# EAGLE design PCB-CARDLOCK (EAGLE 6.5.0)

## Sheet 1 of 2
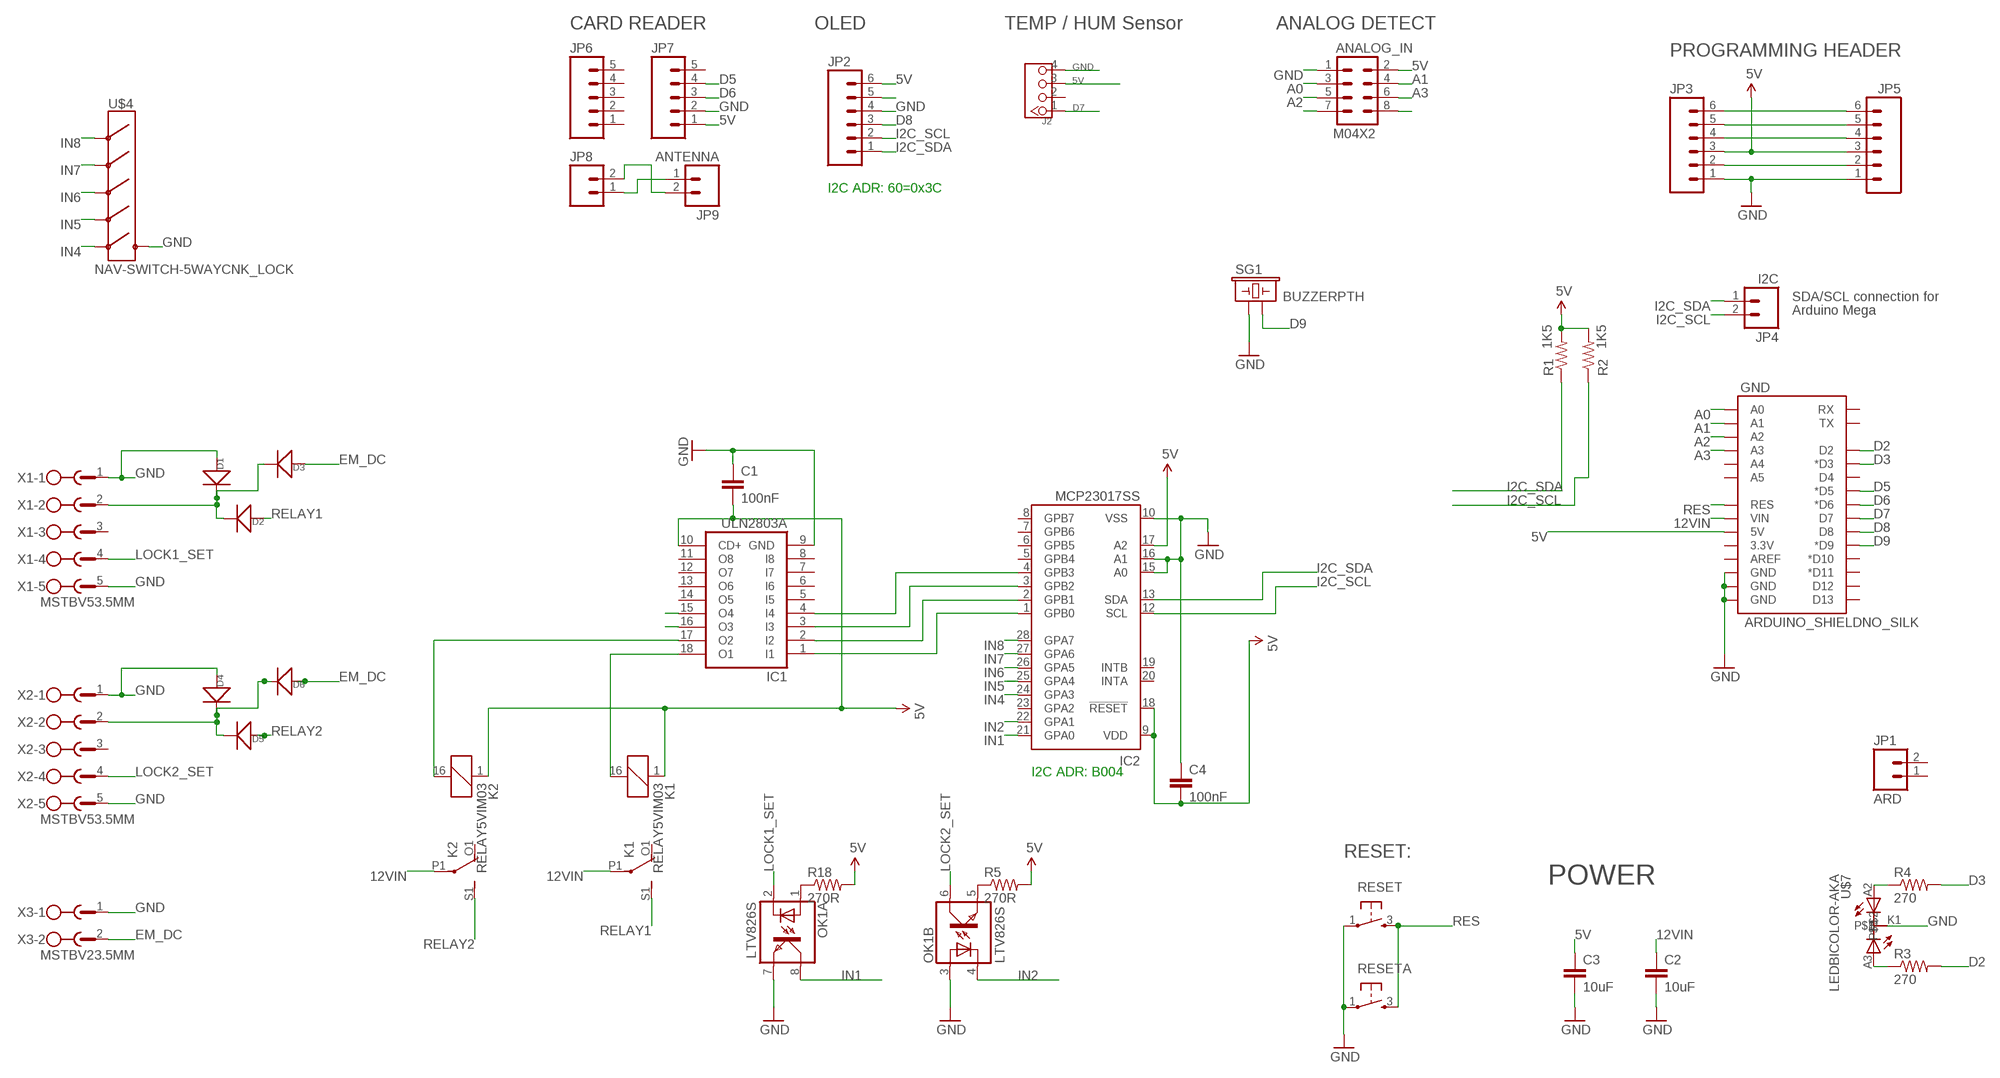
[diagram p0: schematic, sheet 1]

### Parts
ANALOG_IN  M04X2  [2X4]
C1  100nF  CAP0805  [0805]
C2  10uF  CAP0805  [0805]
C3  10uF  CAP0805  [0805]
C4  100nF  CAP0603-CAP  [0603-CAP]
D1  D-SMA  [DO-214AC]
D2  D-SMA  [DO-214AC]
D3  D-SMA  [DO-214AC]
D4  D-SMA  [DO-214AC]
D5  D-SMA  [DO-214AC]
D6  D-SMA  [DO-214AC]
GND  ARDUINO_SHIELDNO_SILK  [DUEMILANOVE_VIAS]
IC1  ULN2803A  ULN2803ASO18W  [SO18W]
IC2  MCP23017SS  [SSOP28]
J2  TWIG-4P-2.0-2.0  [4P-2.0]
JP1  ARD  M02PTH  [1X02]
JP2  M06POLAR  [MOLEX-1X6]
JP3  M06POLAR  [MOLEX-1X6]
JP4  I2C  M02PTH  [1X02]
JP5  M06POLAR  [MOLEX-1X6]
JP6  M05PTH  [1X05]
JP7  M05PTH  [1X05]
JP8  M02PTH  [1X02]
JP9  ANTENNA  M02PTH  [1X02]
K1  RELAY5VIM03  [DS2Y]
K2  RELAY5VIM03  [DS2Y]
OK1  LTV826S  [DIL8-SMD]
R1  1K5  RESISTOR0603-RES  [0603-RES]
R2  1K5  RESISTOR0603-RES  [0603-RES]
R3  270  RESISTOR0603-RES  [0603-RES]
R4  270  RESISTOR0603-RES  [0603-RES]
R5  270R  RESISTOR0603-RES  [0603-RES]
R18  270R  RESISTOR0603-RES  [0603-RES]
RESET  TAC_SWITCH  [PUSHBUTTON]
RESETA  TAC_SWITCH  [PUSHBUTTON]
SG1  BUZZERPTH  [BUZZER-12MM]
U$4  NAV-SWITCH-5WAYCNK_LOCK  [NAV-SWITCH-5WAY]
U$7  LEDBICOLOR-AKA  [LED5MM-BICOLOR]
X1  MSTBV53.5MM  [MSTBV5-3.5]
X2  MSTBV53.5MM  [MSTBV5-3.5]
X3  MSTBV23.5MM  [MSTBV2-3.5]

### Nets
5V [PWR]: ANALOG_IN.2 C1.2 C3.1 C4.2 GND.5V IC1.10(CD+) IC2.9(VDD) IC2.17(A2) IC2.18(!RESET) J2.3 JP2.6 JP3.3 JP5.3 JP7.1 K1.1 K2.1 R1.2 R2.2 R5.2 R18.2
12VIN [PWR]: C2.1 GND.VIN K1.P1(2:P) K2.P1(2:P)
A0: ANALOG_IN.3 GND.A0
A1: ANALOG_IN.4 GND.A1
A2: ANALOG_IN.5 GND.A2
A3: ANALOG_IN.6 GND.A3
D2: GND.D2 R3.2
D3: GND.D3(*D3) R4.2
D5: GND.D5(*D5) JP7.4
D6: GND.D6(*D6) JP7.3
D7: GND.D7 J2.1
D8: GND.D8 JP2.3
D9: GND.D9(*D9) SG1.-
EM_DC [RELAY LINES]: D3.1(+) D6.1(+) X3.2
GND [PWR]: ANALOG_IN.1 C1.1 C2.2 C3.2 C4.1 D1.1(+) D4.1(+) GND.GND@0(GND) GND.GND@1(GND) GND.GND@2(GND) IC1.9(GND) IC2.10(VSS) IC2.15(A0) IC2.16(A1) J2.4 JP2.4 JP3.1 JP5.1 JP7.2 OK1.3(B:A) OK1.7(A:EMIT) RESET.1 RESETA.1 SG1.+ U$4.PIN4(COMMON) U$7.K1 X1.1 X1.5 X2.1 X2.5 X3.1
I2C_SCL: IC2.12(SCL) JP2.2 JP4.2 R2.1
I2C_SDA: IC2.13(SDA) JP2.1 JP4.1 R1.1
IN1: IC2.21(GPA0) OK1.8(A:COL)
IN2: IC2.22(GPA1) OK1.4(B:C)
IN4: IC2.24(GPA3) U$4.PIN6(PUSH)
IN5: IC2.25(GPA4) U$4.PIN5(RIGHT)
IN6: IC2.26(GPA5) U$4.PIN2(LEFT)
IN7: IC2.27(GPA6) U$4.PIN3(DWN)
IN8: IC2.28(GPA7) U$4.PIN1(UP)
LOCK1_SET [PWR]: OK1.2(A:C) X1.4
LOCK2_SET [PWR]: OK1.6(B:COL) X2.4
N$1 [RELAY LINES]: D1.2(-) D2.2(-) D3.2(-) X1.2
N$2: JP8.1 JP9.1
N$3: JP3.4 JP5.4
N$4: IC1.18(O1) K1.16
N$5 [RELAY LINES]: D4.2(-) D5.2(-) D6.2(-) X2.2
N$6: IC1.1(I1) IC2.1(GPB0)
N$7: R4.1 U$7.A2
N$8: JP3.5 JP5.5
N$9: IC1.17(O2) K2.16
N$10: JP8.2 JP9.2
N$11: R3.1 U$7.A3
N$12: JP3.2 JP5.2
N$13: IC1.2(I2) IC2.2(GPB1)
N$14: IC1.3(I3) IC2.3(GPB2)
N$15: JP2.5
N$16: IC1.4(I4) IC2.4(GPB3)
N$17: ANALOG_IN.8
N$18: OK1.5(B:EMIT) R5.1
N$21: ANALOG_IN.7
N$23: OK1.1(A:A) R18.1
N$25: IC1.16(O3)
N$26: IC1.15(O4)
N$45: JP3.6 JP5.6
RELAY1 [RELAY LINES]: D2.1(+) K1.S1(2:S)
RELAY2 [RELAY LINES]: D5.1(+) K2.S1(2:S)
RES: GND.RES RESET.3 RESETA.3
Unconnected: GND.3.3V GND.A4 GND.A5 GND.AREF GND.D4 GND.D10(*D10) GND.D11(*D11) GND.D12 GND.D13 GND.RX GND.TX IC1.5(I5) IC1.6(I6) IC1.7(I7) IC1.8(I8) IC1.11(O8) IC1.12(O7) IC1.13(O6) IC1.14(O5) IC2.5(GPB4) IC2.6(GPB5) IC2.7(GPB6) IC2.8(GPB7) IC2.19(INTB) IC2.20(INTA) IC2.23(GPA2) J2.2 JP1.1 JP1.2 JP6.1 JP6.2 JP6.3 JP6.4 JP6.5 JP7.5 K1.O1(2:O) K1.O2(3:O) K1.P2(3:P) K1.S2(3:S) K2.O1(2:O) K2.O2(3:O) K2.P2(3:P) K2.S2(3:S) X1.3 X2.3

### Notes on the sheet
- CARD READER | OLED | TEMP / HUM Sensor | ANALOG DETECT
- PROGRAMMING HEADER
- I2C ADR: 60=0x3C
- SDA/SCL connection for
- Arduino Mega
- I2C ADR: B004
- RESET:
- POWER

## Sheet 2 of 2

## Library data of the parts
ANALOG_IN = SparkFun:M04X2
C1-C4 = SparkFun:CAP: Capacitor
D1-D6 = OPL:D*: DIODE
GND = SparkFun:ARDUINO_SHIELD
IC1 = uln-udn:ULN2803A: DRIVER ARRAY
IC2 = microchip:MCP23017: http://ww1.microchip.com/downloads/en/DeviceDoc/21952a.pdf Source: http://ww1.microchip.com/downloads/en/DeviceDoc/21952a.pdf; MF: MICROCHIP; MPN: MCP23017-E/SS; OC_FARNELL: 1467674; OC_NEWARK: 31K2960
J2 = Connector :TWIG-4P-2.0
JP1 JP4 JP8 JP9 = SparkFun:M02: Header 2
JP2 JP3 JP5 = SparkFun:M06: Header 6 Standard 6-pin 0.1" header. Use with straight break away headers (SKU : PRT-00116), right angle break away headers (PRT-00553), swiss pins (PRT-00743), machine pins (PRT-00117), and female headers (PRT-00115). Molex polarized connector foot print use with SKU : PRT-08094 with associated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
JP6 JP7 = SparkFun:M05: Header 5 Standard 5-pin 0.1" header. Use with straight break away headers (SKU : PRT-00116), right angle break away headers (PRT-00553), swiss pins (PRT-00743), machine pins (PRT-00117), and female headers (PRT-00115). Molex polarized connector foot print use with SKU : PRT-08230 with associated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
K1 K2 = SKAARHOJ:RELAY5V: RELAY 2 x switch, AxiCom 150 mW 5V
OK1 = optocoupler:LTV826: OPTO COUPLER Source: LITEON, LTV816.pdf; OC_FARNELL: unknown; OC_NEWARK: unknown
R1-R5 R18 = SparkFun:RESISTOR: Resistor
RESET RESETA = SKAARHOJ:TAC_SWITCH: Momentary Switch
SG1 = SparkFun:BUZZER: Buzzer 12mm
U$4 = SKAARHOJ:NAV-SWITCH-5WAY: For use with a push-button switch made by CnK components. The Part # is
U$7 = SKAARHOJ:LEDBICOLOR-AKA
X1 X2 = SKAARHOJ:MSTBV5: PHOENIX
X3 = SKAARHOJ:MSTBV2: PHOENIX

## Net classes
0 default: width 0.203 mm, drill 0.406 mm, clearance 0.203 mm
1 PWR: width 0.406 mm, drill 0.61 mm, clearance 0.203 mm
2 RELAY LINES: width 0.305 mm, clearance 0.203 mm
3 INput lines: clearance 0.203 mm

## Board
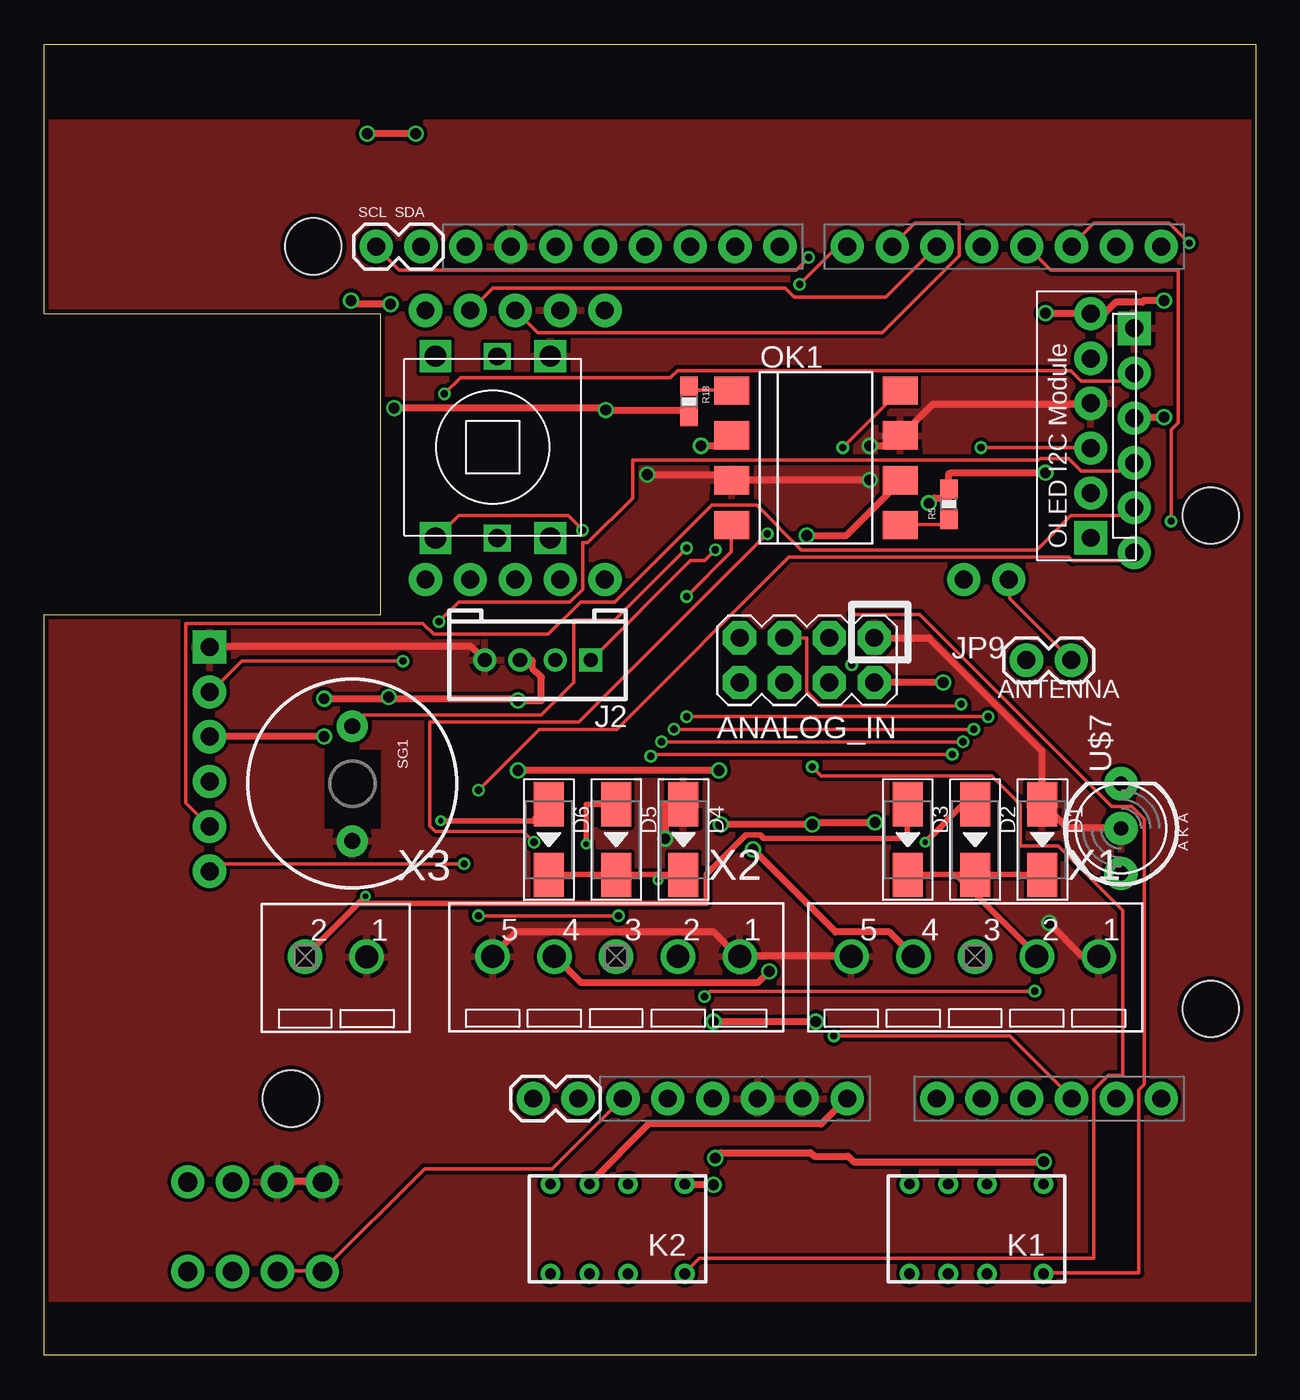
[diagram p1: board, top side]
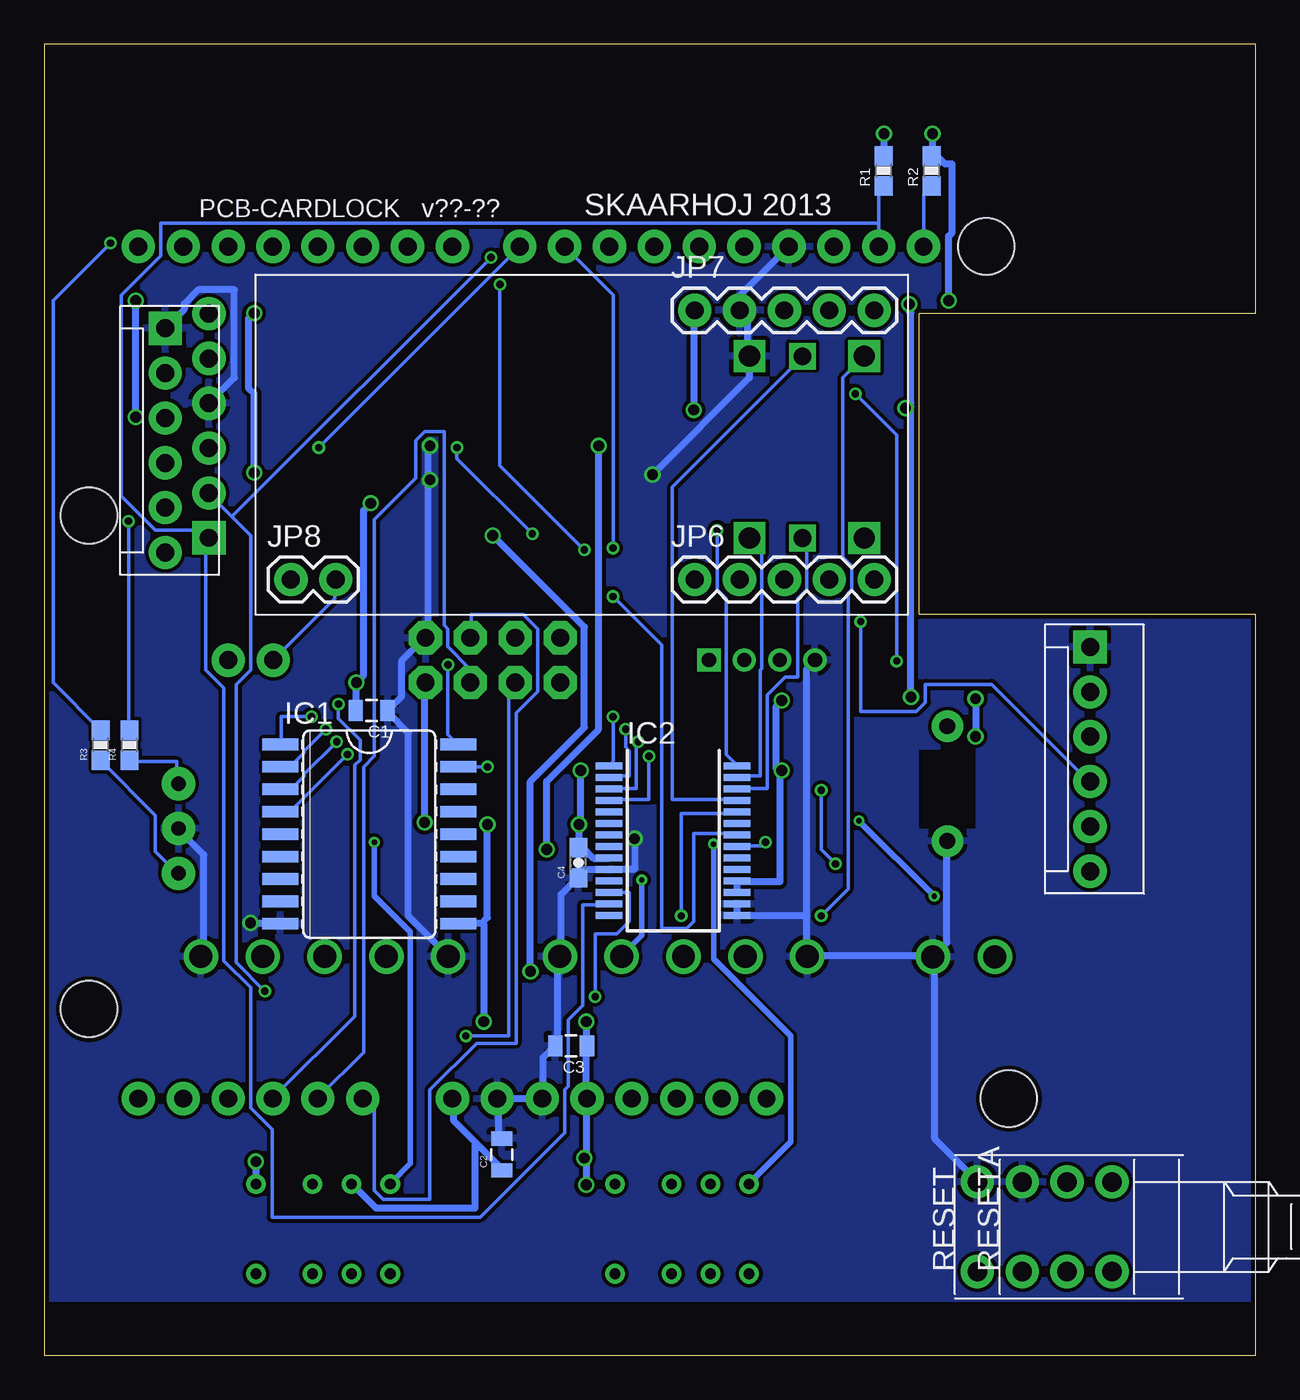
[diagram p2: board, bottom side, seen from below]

Size 68.58 x 74.26 mm. Coordinates in mm from the lower left corner, seen from the top.
Outline: 0,0 0,41.96 19.05,41.96 19.05,58.99 0,58.99 0,74.26 68.58,74.26 68.58,0 0,0
Copper layers (1*16): Top 0.035mm / dielectric 1.5mm / Bottom 0.035mm
Design rules "Fusion_eagle_rule_v1.1": minimum track width 6mil, minimum drill 12mil, track to track 6mil, track to pad 6mil, pad to pad 6mil, via to via 6mil, smd to smd 0mil, copper to edge 10mil, drill to drill 10mil, minimum pad ring 10mil, minimum via ring 6mil, stop-mask expansion 2mil, vias tented up to drill 100mil, thermal gap 10mil
Holes 3.2 mm at 66.04,47.56 15.24,62.8 13.97,14.54 66.04,19.62
tRestrict: area 0,0 to 68.6,3; area 0,70 to 68.6,74; area 15.9,29.8 to 19,34.3
bRestrict: area 0,70 to 68.6,74; area 0,0 to 68.6,3; area 15.9,29.8 to 19,34.3

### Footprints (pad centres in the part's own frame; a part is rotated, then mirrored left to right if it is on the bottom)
2X4 = drill 1.016 pad 1.88 octagon: 1 -3.81,-1.27; 2 -3.81,1.27; 3 -1.27,-1.27; 4 -1.27,1.27; 5 1.27,-1.27; 6 1.27,1.27; 7 3.81,-1.27; 8 3.81,1.27
0805 = smd 0.8 x 1.2: 1 -0.9,0; 2 0.9,0
0603-CAP = smd 1.1 x 1: 1 -0.85,0; 2 0.85,0
DO-214AC = smd 2.5 x 1.7: 1 -2,0; 2 2,0
DUEMILANOVE_VIAS = drill 1.016 pad 1.88: 3.3V 50.8,13.97; 5V 50.8,16.51; A0 50.8,29.21; A1 50.8,31.75; A2 50.8,34.29; A3 50.8,36.83; A4 50.8,39.37; A5 50.8,41.91; AREF 2.54,2.54; D2 2.54,36.83; D3 2.54,34.29; D4 2.54,31.75; D5 2.54,29.21; D6 2.54,26.67; D7 2.54,24.13; D8 2.54,20.32; D9 2.54,17.78; D10 2.54,15.24; D11 2.54,12.7; D12 2.54,10.16; D13 2.54,7.62; GND@0 50.8,19.05; GND@1 50.8,21.59; GND@2 2.54,5.08; RES 50.8,11.43; RX 2.54,41.91; TX 2.54,39.37; VIN 50.8,24.13
SO18W = smd 0.66 x 2.032: 1 -5.08,-5.029; 2 -3.81,-5.029; 3 -2.54,-5.029; 4 -1.27,-5.029; 5 0,-5.029; 6 1.27,-5.029; 7 2.54,-5.029; 8 3.81,-5.029; 9 5.08,-5.029; 10 5.08,5.029; 11 3.81,5.029; 12 2.54,5.029; 13 1.27,5.029; 14 0,5.029; 15 -1.27,5.029; 16 -2.54,5.029; 17 -3.81,5.029; 18 -5.08,5.029
SSOP28 = smd 0.4 x 1.5: 1 -4.225,-3.625; 2 -3.575,-3.625; 3 -2.925,-3.625; 4 -2.275,-3.625; 5 -1.625,-3.625; 6 -0.975,-3.625; 7 -0.325,-3.625; 8 0.325,-3.625; 9 0.975,-3.625; 10 1.625,-3.625; 11 2.275,-3.625; 12 2.925,-3.625; 13 3.575,-3.625; 14 4.225,-3.625; 15 4.225,3.625; 16 3.575,3.625; 17 2.925,3.625; 18 2.275,3.625; 19 1.625,3.625; 20 0.975,3.625; 21 0.325,3.625; 22 -0.325,3.625; 23 -0.975,3.625; 24 -1.625,3.625; 25 -2.275,3.625; 26 -2.925,3.625; 27 -3.575,3.625; 28 -4.225,3.625
4P-2.0 = drill 0.8 pad 1.27 square: 1 -3,0 | drill 0.8 pad 1.27: 2 -1,0; 3 1,0; 4 3,0
1X02 = drill 1.016 pad 1.88: 1 0,0; 2 2.54,0
MOLEX-1X6 = drill 1.016 pad 1.88 square: 1 0,0 | drill 1.016 pad 1.88: 2 2.54,0; 3 5.08,0; 4 7.62,0; 5 10.16,0; 6 12.7,0
1X05 = drill 1.016 pad 1.88: 1 0,0; 2 2.54,0; 3 5.08,0; 4 7.62,0; 5 10.16,0
DS2Y = drill 0.6: 1 1.2,0.46; 16 1.2,5.54; O1 4.4,0.46; O2 4.4,5.54; P1 6.6,0.46; P2 6.6,5.54; S1 8.8,0.46; S2 8.8,5.54
DIL8-SMD = smd 1.6 x 2: 1 -3.81,-4.77; 2 -1.27,-4.77; 3 1.27,-4.77; 4 3.81,-4.77; 5 3.81,4.77; 6 1.27,4.77; 7 -1.27,4.77; 8 -3.81,4.77
0603-RES = smd 1.1 x 1: 1 -0.85,0; 2 0.85,0
PUSHBUTTON = drill 1.1 pad 1.88: 1 2.54,2.54; 2 2.54,-2.54; 3 -2.54,2.54; 4 -2.54,-2.54
BUZZER-12MM = drill 0.9 pad 1.778: + 3.25,0; - -3.25,0
NAV-SWITCH-5WAY = drill 1.2 square: PIN1 -5.15,3.25; PIN3 -5.15,-3.25; PIN4 5.15,-3.25; PIN6 5.15,3.25 | drill 1 square: PIN2 -5.15,-0.25; PIN5 5.15,-0.25
LED5MM-BICOLOR = drill 0.813 pad 1.88: A2 2.54,0; A3 -2.54,0; K1 0,0
MSTBV5-3.5 = drill 1.3: 1 -7,0; 2 -3.5,0; 3 0,0; 4 3.5,0; 5 7,0
MSTBV2-3.5 = drill 1.3: 1 -1.75,0.02; 2 1.75,0.02

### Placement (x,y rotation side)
ANALOG_IN  43.18,39.37 180 top
C1  50.04,36.52 180 bottom
C2  42.67,11.38 90 bottom
C3  38.75,17.53 180 bottom
C4  38.34,27.89 90 bottom
D1  56.52,29.21 270 top
D2  52.7,29.21 270 top
D3  48.9,29.21 270 top
D4  36.2,29.21 270 top
D5  32.38,29.21 270 top
D6  28.57,29.21 270 top
GND  21.34,65.34 270 top
IC1  50.17,29.52 270 bottom
IC2  32.97,29.14 270 bottom
J2  27.94,39.37 180 top
JP1  27.69,14.54 0 top
JP2  59.25,46.3 90 top
JP3  61.72,58.17 270 bottom
JP4  21.34,62.8 180 top
JP5  9.36,40.12 270 bottom
JP6  31.75,43.94 0 bottom
JP7  31.75,59.18 0 bottom
JP8  54.61,43.94 0 bottom
JP9  58.15,39.37 180 top
K1  57.78,10.16 180 top
K2  37.47,10.16 180 top
OK1  43.7,50.83 270 top
R1  21.05,67.09 90 bottom
R2  18.33,67.09 90 bottom
R3  65.38,34.56 90 bottom
R4  63.74,34.56 90 bottom
R5  51.23,48.21 90 top
R18  36.5,54.02 270 top
RESET  13.21,7.29 90 bottom
RESETA  10.67,7.29 90 bottom
SG1  17.45,32.38 270 top
U$4  25.4,51.44 90 top
U$7  60.97,29.84 90 top
X1  52.7,22.59 180 top
X2  32.38,22.59 180 top
X3  16.51,22.59 180 top

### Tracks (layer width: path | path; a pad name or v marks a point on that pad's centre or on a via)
5V  (via drill 0.61)
  Top 0.406: v63.4,59.74 62.28,59.74 62.18,59.64 60.66,59.64 60.05,59.03 59.33,59.03 JP2.6 59.13,59.03 v56.69,59.03 | v63.4,53.14 61.77,53.14 JP3.3 | v50.9,38.1 ANALOG_IN.2 | v50.09,48.26 50.39,48.56 51.21,48.56 51.21,48.97 R5.2 51.21,49.17 51.21,49.89 51.31,49.99 v56.69,49.99 | v21.03,69.19 v18.29,69.19 | R18.2 36.47,53.24 36.47,53.54 v31.8,53.54 31.7,53.65 v19.81,53.65 | v17.37,59.74 17.58,59.54 v19.61,59.54 | v37.9,9.65 36.27,9.65 K2.1 | v56.59,10.97 45.82,10.97 45.52,11.28 43.59,11.28 43.38,11.48 38.3,11.48 v38,11.18 | v38.3,30.07 v43.48,30.07 43.59,30.18 v47.04,30.18 | v38.2,33.12 v26.82,33.12 | J2.3 27.03,39.42 27.53,39.42 27.64,39.32 27.64,38.91 28.14,38.41 28.14,37.08 v26.82,37.08 26.72,37.19 19.51,37.19 | v15.85,35.05 9.45,35.05 JP5.3 | 19.51,37.19 v15.85,37.19 | v43.69,18.9 v37.9,18.9 | v19.51,37.29 19.51,37.19
  Bottom 0.406: v63.4,53.14 v63.4,59.74 | C1.2 50.9,36.58 v50.9,38.1 50.49,38.51 50.49,47.85 v50.09,48.26 | v56.69,59.03 57,58.73 57,54.76 56.69,54.46 v56.69,49.99 | v18.29,69.19 18.29,67.97 R2.2 18.09,67.97 17.58,67.46 17.17,67.46 17.17,63.6 17.37,63.4 v17.37,59.74 | v21.03,69.19 21.03,67.97 R1.2 | v31.8,53.54 31.8,59.13 JP7.1 | v19.61,59.54 19.61,59.13 19.51,59.03 19.51,53.95 v19.81,53.65 19.51,53.75 v19.51,37.29 | 37.9,11.18 37.9,14.43 GND.5V 37.9,14.63 37.9,17.48 C3.1 37.9,17.68 v37.9,18.9 | 37.9,11.18 v37.9,9.65 | v56.59,10.97 56.59,9.75 K1.1 | v38,11.18 37.9,11.18 | IC2.17 29.36,26.31 29.36,26.82 IC2.18 29.16,26.82 26.92,26.82 26.92,33.02 v26.82,33.12 27.03,33.12 27.13,33.22 27.13,36.78 v26.82,37.08 | v43.48,30.07 43.48,24.79 43.79,24.49 | 43.79,24.49 45.11,24.49 IC1.10 | IC2.9 36.68,28.14 37.49,28.14 38.1,28.75 C4.2 38.3,28.75 v38.3,30.07 38.2,30.18 v38.2,33.12 | v15.85,37.19 v15.85,35.05 | v43.69,18.9 43.69,24.38 43.79,24.49 | v47.04,30.18 47.04,38.1 ANALOG_IN.2
12VIN
  Top 0.406: K2.P1 30.89,9.75 34.24,13.11 43.99,13.11 45.41,14.53 GND.VIN
  Bottom 0.406: 44.09,11.99 45.41,13.31 45.41,14.53 GND.VIN | 44.09,11.99 42.67,10.57 C2.1 | K1.P1 51.1,9.65 49.78,8.33 44.2,8.33 44.2,11.89 44.09,11.99
A0
  Bottom 0.203: GND.A0 50.49,14.53 49.89,13.92 49.89,9.35 49.38,8.84 46.74,8.84 46.74,15.04 44.09,17.68 41.86,17.68 41.86,36.37 40.64,37.59 40.64,41.15 41.45,41.96 44.4,41.96 44.4,40.64 ANALOG_IN.3
A1
  Bottom 0.203: GND.A1 53.03,14.63 50.49,17.17 50.49,33.33 49.89,33.93 49.89,47.35 47.55,49.68 47.55,51.82 47.04,52.32 45.92,52.32 45.92,41.35 45.72,41.15 45.72,40.13 44.5,38.91 44.5,38.1 ANALOG_IN.4
A2  (via drill 0.41)
  Top 0.203: v51.92,36.88 51.82,36.78 43.99,36.78 43.18,37.59 43.18,40.64 ANALOG_IN.5
  Bottom 0.203: v51.92,36.88 51.92,36.07 50.7,34.85 50.7,33.73 51,33.43 51,19.2 55.58,14.63 GND.A2
A3  (via drill 0.41)
  Top 0.203: v44.7,18.09 54.66,18.09 58.12,14.63 GND.A3
  Bottom 0.203: v44.7,18.09 42.27,18.09 42.27,37.8 41.96,38.1 ANALOG_IN.6
D2  (via drill 0.41)
  Top 0.203: v64.82,62.99 63.7,64.11 59.44,64.11 58.22,62.89 GND.D2
  Bottom 0.203: v64.82,62.99 68.07,59.74 68.07,38.1 65.43,35.46 R3.2
D3  (via drill 0.41)
  Top 0.203: v63.8,47.24 63.8,52.43 64.21,52.83 64.21,61.47 57,61.47 55.68,62.79 GND.D3
  Bottom 0.203: v63.8,47.24 63.8,35.46 R4.2
D5
  Top 0.203: JP7.4 25.4,60.45 41.96,60.45 42.47,59.94 47.65,59.94 50.49,62.79 GND.D5
D6
  Top 0.203: JP7.3 27.94,57.91 47.45,57.91 51.82,62.28 51.82,64.11 49.28,64.11 48.06,62.89 GND.D6
D7  (via drill 0.41)
  Top 0.203: v38,45.62 37.39,45.01 36.58,45.01 30.99,39.42 J2.1 | v42.77,60.66 44.91,62.79 45.41,62.79 GND.D7
  Bottom 0.203: v38,45.62 42.77,50.39 v42.77,60.66
D8  (via drill 0.41)
  Top 0.203: v53.03,51.41 59.23,51.41 JP2.3
  Bottom 0.203: v53.03,51.41 GND.D8
D9  (via drill 0.41)
  Top 0.203: v36.37,45.72 32.31,41.66 29.97,41.66 29.97,38.1 28.14,36.27 18.09,36.27 17.48,35.66 SG1.-
  Bottom 0.203: v36.37,45.72 36.37,60.05 GND.D9
EM_DC  (via drill 0.3)
  Top 0.305: v22.45,30.28 27.64,30.28 28.55,31.19 D6.1 | 17.88,25.7 14.83,22.66 X3.2 | 17.88,25.7 v18.19,26.01 | D3.1 48.87,31.19 48.87,29.26 40.74,29.26 40.54,29.46 39.73,29.46 37.49,27.23 37.49,25.6 17.98,25.6 17.88,25.7
  Bottom 0.305: v18.19,26.01 v22.45,30.28
GND  (via drill 0.61)
  Top 0.406: RESETA.1 13.21,9.86 15.75,9.86 RESET.1 | JP5.1 9.45,40.13 24.18,40.13 24.89,39.42 J2.4 | v34.14,49.89 38.61,49.89 38.91,49.58 OK1.3 39.12,49.58 v46.74,49.58 | JP2.4 59.23,53.85 50.29,53.85 48.56,52.12 OK1.7 48.26,52.12 47.65,51.51 v46.74,51.51 | U$7.K1 60.96,29.87 57.91,29.87 56.59,31.19 D1.1 56.49,31.39 56.49,34.24 50.09,40.64 ANALOG_IN.1 | v56.9,24.49 58.73,22.66 59.64,22.66 X1.1 | v35.15,29.26 35.15,31.19 36.17,31.19 D4.1 | X1.5 45.62,22.66 39.42,22.66 X2.1 39.22,22.66 37.9,23.98 26.72,23.98 25.4,22.66 X2.5
  Bottom 0.406: SG1.+ 17.48,29.06 17.48,23.37 18.19,22.66 X3.1 | RESET.1 15.75,9.86 18.19,12.29 18.19,22.45 X3.1 | IC2.16 29.36,25.5 29.36,24.99 IC2.15 29.16,24.89 25.4,24.89 | 25.4,24.89 25.4,22.66 X2.5 25.2,22.66 18.39,22.66 X3.1 | 25.4,24.89 25.4,38.91 24.99,39.32 J2.4 | v34.14,49.89 28.65,55.37 28.65,56.49 U$4.PIN4 28.75,56.69 28.75,58.73 JP7.2 29.16,59.33 29.16,60.05 GND.GND@2 | JP3.1 60.66,59.23 60.66,59.54 59.84,60.35 57.81,60.35 57.81,55.37 59.23,53.95 JP2.4 | v56.9,24.49 55.27,24.49 IC1.9 | U$7.K1 60.96,29.77 59.54,28.35 59.54,22.76 59.64,22.66 X1.1 | C2.2 42.67,12.29 42.88,12.5 42.88,14.53 GND.GND@1 42.67,14.53 40.54,14.53 GND.GND@0 40.34,14.63 40.34,16.87 39.73,17.48 C3.2 39.52,17.68 39.52,22.45 X2.1 39.32,22.66 39.32,26.11 38.41,27.03 C4.1 38.3,27.23 38.3,27.53 36.78,27.53 IC2.10 36.58,27.53 35.15,27.53 v35.15,29.26 | X1.5 45.72,22.66 47.95,24.89 47.95,35.26 49.07,36.37 C1.1 49.07,36.58 48.36,37.29 48.36,39.32 47.04,40.64 ANALOG_IN.1 46.84,40.74 46.84,49.58 | v46.74,51.51 46.84,51.41 46.84,49.58 | v46.74,49.58 46.84,49.58
  pour Top: 0,0 68.58,0 68.58,74.3 0,74.3
  pour Bottom: 0,0 68.58,0 68.58,74.3 0,74.3
I2C_SCL  (via drill 0.41)
  Top 0.203: v37.39,20.32 37.69,20.62 v56.08,20.62 | v43.28,62.18 42.57,61.47 20.12,61.47 JP4.2
  Bottom 0.203: JP4.2 18.8,65.73 18.39,66.14 R2.1 | v37.39,20.32 37.39,23.88 36.17,23.88 35.46,24.59 35.46,26.21 36.58,26.21 IC2.12 | v56.08,20.62 57.71,22.25 57.71,38 56.9,38.81 56.9,46.43 57.96,47.5 | 57.96,47.5 59.23,48.77 JP2.2 | 57.96,47.5 v43.28,62.18
I2C_SDA
  Bottom 0.203: JP4.1 21.34,64.11 | 21.34,64.11 21.34,65.94 21.13,66.14 R1.1 | IC2.13 36.68,25.5 38.1,25.5 38.1,19.81 38.91,19 38.91,15.24 39.12,15.04 39.12,12.6 43.89,7.82 55.68,7.82 55.68,12.8 56.9,14.02 56.9,20.83 58.42,22.35 58.42,37.8 59.44,38.81 59.44,46.13 59.33,46.23 JP2.1 59.33,46.33 59.33,46.74 62.28,46.74 64.21,48.67 64.21,60.05 61.98,62.28 61.98,64.11 21.34,64.11
IN1  (via drill 0.41)
  Top 0.203: v27.74,29.06 27.13,29.67 22.15,29.67 21.84,29.97 21.84,35.87 30.28,35.87 v40.95,46.53 | v45.21,51.41 48.36,54.56 48.46,54.56 OK1.8
  Bottom 0.203: v27.74,29.06 27.74,28.85 29.26,28.85 IC2.21 | v40.95,46.53 45.21,50.8 v45.21,51.41
IN2  (via drill 0.41)
  Top 0.203: v36.37,42.98 38.91,45.52 38.91,46.94 OK1.4
  Bottom 0.203: v36.37,42.98 33.63,40.23 33.63,24.18 32.21,24.18 31.8,24.59 31.8,29.57 29.36,29.57 IC2.22
IN4  (via drill 0.41)
  Top 0.203: v24.59,24.89 v32.51,24.89
  Bottom 0.203: v32.51,24.89 32.51,30.68 29.36,30.68 IC2.24 | v24.59,24.89 23.06,26.42 23.06,43.18 22.86,43.38 22.86,44.7 23.37,45.21 23.37,55.37 22.25,56.49 U$4.PIN6
IN5
  Bottom 0.203: IC2.25 29.36,31.5 33.02,31.5 33.02,49.17 25.7,56.49 U$4.PIN5
IN6
  Bottom 0.203: IC2.26 29.26,32.11 27.64,32.11 27.64,37.39 26.62,38.41 25.91,38.41 25.91,42.88 25.4,43.38 25.4,46.02 25.6,46.23 U$4.PIN2
IN7
  Bottom 0.203: IC2.27 29.26,32.82 28.04,32.82 28.04,38.81 27.94,38.91 27.94,45.62 28.55,46.23 U$4.PIN3
IN8  (via drill 0.41)
  Top 0.203: v30.48,46.74 29.67,47.55 23.47,47.55 22.25,46.33 U$4.PIN1
  Bottom 0.203: v30.48,46.74 30.48,43.38 29.97,42.88 29.97,34.04 29.36,33.43 IC2.28
LOCK1_SET  (via drill 0.61)
  Top 0.406: v37.19,51.51 38.41,51.51 38.91,52.02 OK1.2 | v40.13,28.65 44.81,23.98 47.85,23.98 49.17,22.66 X1.4
  Bottom 0.406: v37.19,51.51 37.19,35.46 40.13,32.51 v40.13,28.65
LOCK2_SET  (via drill 0.61)
  Top 0.406: v43.18,46.43 45.41,46.43 48.46,49.48 OK1.6 | v41.05,21.74 40.44,21.13 30.38,21.13 28.96,22.55 X2.4
  Bottom 0.406: v43.18,46.43 38,41.25 38,35.56 41.05,32.51 v41.05,21.74
N$1
  Top 0.305: 51.71,27.23 52.63,27.23 D2.2 52.83,27.23 56.49,27.23 D1.2 | 51.71,27.23 48.97,27.23 D3.2 | X1.2 56.19,22.66 51.71,27.13 51.71,27.23
N$2
  Top 0.203: JP9.1 58.12,39.42 54.66,42.88 54.66,43.89 JP8.1
N$3  (via drill 0.41)
  Top 0.203: v22.35,41.55 23.47,42.67 29.77,42.67 30.48,43.38 30.48,46.02 30.79,46.02 33.33,48.56 33.33,50.7 56.29,50.7 56.39,50.8 58.01,50.8 58.73,50.09 61.27,50.09 JP3.4
  Bottom 0.203: v22.35,41.55 22.35,36.47 19.2,36.47 18.69,36.98 18.69,38 14.94,38 9.45,32.51 JP5.4
N$4  (via drill 0.41)
  Top 0.203: v45.72,39.12 45.72,41.96 49.58,41.96 60.45,31.09 61.57,31.09 62.28,30.38 62.28,15.34 61.98,15.04 61.98,4.67 56.59,4.67 K1.16
  Bottom 0.203: v45.72,39.12 45.72,35.15 45.21,34.65 IC1.18
N$5  (via drill 0.3)
  Top 0.305: D6.2 28.65,27.23 32.31,27.23 D5.2 32.51,27.23 34.75,27.23 | 34.75,27.23 36.17,27.23 D4.2 | 34.75,27.23 v34.75,26.92
  Bottom 0.305: v34.75,26.92 34.75,23.77 35.87,22.66 X2.2
N$6  (via drill 0.41)
  Top 0.203: v53.44,36.17 v36.37,36.17
  Bottom 0.203: v36.37,36.17 36.37,33.63 36.58,33.43 IC2.1 | v53.44,36.17 55.17,36.17 55.17,34.65 IC1.1
N$7
  Bottom 0.203: R4.1 63.7,33.63 61.06,33.63 61.06,32.41 U$7.A2
N$8
  Top 0.203: JP3.5 61.27,47.55 58.12,47.55 56.19,45.62 42.88,45.62 40.34,48.16 37.8,48.16 32.31,42.67 30.38,42.67 28.55,40.84 22.05,40.84 21.44,41.45 8.03,41.45 8.03,31.29 9.35,29.97 JP5.5
N$9  (via drill 0.41)
  Top 0.203: v43.48,33.33 43.99,32.82 53.65,32.82 55.27,31.19 55.27,28.85 57.4,28.85 61.06,25.2 61.06,15.85 60.25,15.85 59.44,15.04 59.44,5.49 37.08,5.49 36.27,4.67 K2.16
  Bottom 0.203: v43.48,33.33 45.11,33.33 IC1.17
N$10
  Bottom 0.203: JP9.2 55.58,39.42 52.12,42.88 52.12,43.89 JP8.2
N$11
  Bottom 0.203: R3.1 65.33,33.63 62.28,30.58 62.28,28.55 61.06,27.33 U$7.A3
N$12  (via drill 0.41)
  Top 0.203: v20.32,39.32 11.18,39.32 9.45,37.59 JP5.2 | v22.66,54.46 23.57,55.37 35.46,55.37 35.87,55.78 58.12,55.78 58.73,55.17 61.27,55.17 JP3.2
  Bottom 0.203: v20.32,39.32 20.32,52.12 v22.66,54.46
N$13  (via drill 0.41)
  Top 0.203: v52.63,35.46 v35.66,35.46
  Bottom 0.203: v35.66,35.46 35.66,34.44 35.46,34.24 35.46,32.82 36.58,32.82 IC2.2 | v52.63,35.46 53.85,34.24 53.85,34.14 54.56,33.43 55.17,33.43 IC1.2
N$14  (via drill 0.41)
  Top 0.203: v52.02,34.75 v34.95,34.75
  Bottom 0.203: v34.95,34.75 35.05,34.65 35.05,32.11 36.58,32.11 IC2.3 | v52.02,34.75 53.85,32.92 53.85,32.82 54.56,32.11 55.17,32.11 IC1.3
N$16  (via drill 0.41)
  Top 0.203: v34.34,33.93 34.44,34.04 v51.41,34.04
  Bottom 0.203: v34.34,33.93 34.34,31.5 36.58,31.5 IC2.4 | v51.41,34.04 54.56,30.89 55.17,30.89 IC1.4
N$18
  Top 0.203: R5.1 51.21,47.35 50.9,47.04 48.56,47.04 OK1.5
N$23
  Top 0.203: R18.1 36.58,54.86 36.78,54.66 38.91,54.66 OK1.1
N$45  (via drill 0.41)
  Top 0.203: v23.77,27.84 9.86,27.84 9.45,27.43 JP5.6 | v24.59,32 28.04,35.46 32.41,35.46 42.16,45.21 58.01,45.21 58.22,45.01 61.27,45.01 JP3.6
  Bottom 0.203: v23.77,27.84 24.59,28.65 v24.59,32
RELAY1  (via drill 0.3)
  Top 0.305: v49.89,29.06 52.02,31.19 52.63,31.19 D2.1
  Bottom 0.305: v49.89,29.06 49.89,26.01 47.85,23.98 47.85,10.87 48.97,9.75 K1.S1
RELAY2  (via drill 0.3)
  Top 0.305: v30.68,28.96 30.68,31.19 32.31,31.19 D5.1
  Bottom 0.305: v30.68,28.96 30.68,22.45 26.31,18.09 26.31,12.09 28.65,9.75 K2.S1
RES
  Top 0.203: 15.75,4.78 13.21,4.78 RESETA.3 | 15.75,4.78 21.54,10.57 28.75,10.57 32.72,14.53 GND.RES | 15.75,4.78 RESET.3

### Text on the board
_tsilk: SCL SDA | OLED I2C Module | ANTENNA
_bsilk: SKAARHOJ 2013 | PCB-CARDLOCK v??-??

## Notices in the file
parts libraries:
SparkFun: Licensing: CC v3.0 Share-Alike You are welcome to use this library for commercial purposes.
